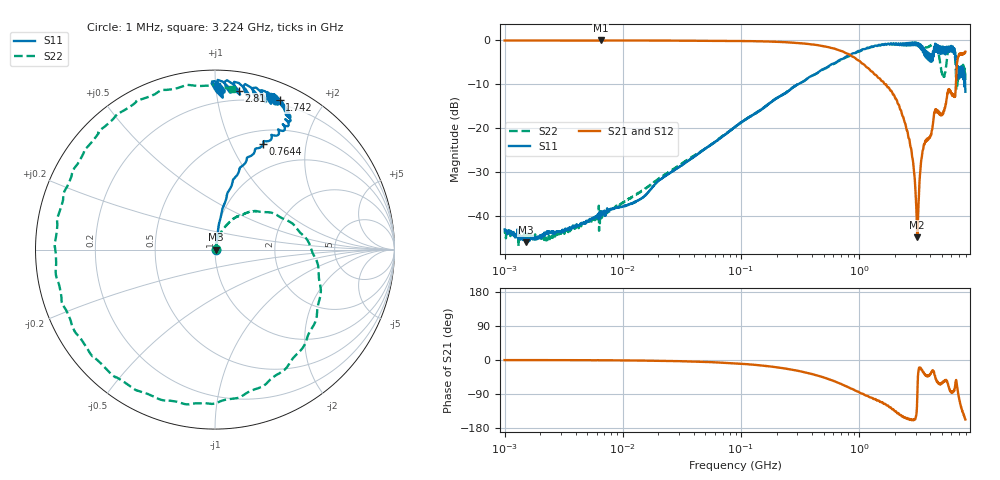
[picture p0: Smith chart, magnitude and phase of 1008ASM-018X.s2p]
!s-Parameter Generated by FASTRON Sdn. Bhd.
!FASTRON P/N : 1008ASM-018X
!Keysight Technologies: E5071C_MY46733604_B.14.02
!Date: Tue Nov 21 11:08:02 2023
!Version  :Rev00  Wed Nov 22 15:46:34 2023
!Data & Calibration Information:
!Freq  S11:SOLT2(ON)  S21:SOLT2(ON)  S12:SOLT2(ON)  S22:SOLT2(ON)
!PortZ  Port1:50+j0  Port2:50+j0
!When reading reference impedance value at option line is always used.
! Remarks : This data is being provided solely for informational purposes.
# Hz S dB R 50
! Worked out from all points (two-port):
!   1599 points, 1 MHz to 7.923 GHz, reference 50 ohm
!   highest |S21| = -0.04 dB at 6.532 MHz (marker M1); lowest = -44.8 dB at 3.102 GHz (marker M2)
!   |S21| within 3 dB of the highest: start of sweep to 795.7 MHz; 7.688 GHz to end of sweep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
!   lowest |S11| = -45.9 dB at 1.505 MHz (marker M3), VSWR 1.01, Z = 50.5 + j0.0493 ohm
!   |S11| at or under -10 dB: start of sweep to 303.3 MHz; 7.79954 GHz to 7.819798 GHz (20.26 MHz wide, 0.259 % of centre); 7.889954 GHz to end of sweep
!   |S22| runs from -46.8 to -0.6 dB; largest |S21 - S12| = 0.013
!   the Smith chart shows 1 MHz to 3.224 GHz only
!   S11 on the Smith chart (normalised r, x): 1 MHz: 1.01, +0.00; 764.4 MHz: 0.66, +1.33; 1.742 GHz: 0.16, +1.51; 2.81 GHz: 0.13, +1.15; 3.224 GHz: 0.09, +1.01
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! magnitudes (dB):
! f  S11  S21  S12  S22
! 1 MHz  -43.0  -0.1  -0.1  -43.4
! 1.505 MHz  -45.9  -0.1  -0.1  -44.7
! 4.479 MHz  -41.5  -0.1  -0.1  -42.0
! 6.532 MHz  -39.1  0.0  -0.1  -38.5
! 19.95 MHz  -32.0  -0.1  -0.1  -31.5
! 89.01 MHz  -19.7  -0.1  -0.2  -19.7
! 398.5 MHz  -8.0  -0.9  -0.9  -8.1
! 764.4 MHz  -3.8  -2.9  -2.9  -4.0
! 1.742 GHz  -0.8  -10.7  -10.7  -0.9
! 1.784 GHz  -0.8  -10.8  -10.8  -0.9
! 2.296 GHz  -1.1  -16.7  -16.7  -1.0
! 2.81 GHz  -1.0  -26.5  -26.5  -0.6
! 3.102 GHz  -1.1  -44.8  -44.8  -0.7
! 3.224 GHz  -0.8  -33.3  -33.3  -0.9
! 3.366 GHz  -2.1  -27.0  -27.0  -1.1
! 3.568 GHz  -3.4  -23.7  -23.7  -1.5
! 4.437 GHz  -1.6  -16.1  -16.2  -0.9
! 5.164 GHz  -3.0  -16.4  -16.4  -8.5
! 5.752 GHz  -2.6  -11.1  -11.1  -1.5
! 6.149 GHz  -2.6  -12.2  -12.2  -2.0
! 6.805 GHz  -6.5  -4.5  -4.5  -9.0
! 7.923 GHz  -11.7  -2.6  -2.6  -9.0
